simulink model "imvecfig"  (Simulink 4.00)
settings: Solver=ode45  StartTime=0.0  StopTime=10.0  RelTol=1e-3
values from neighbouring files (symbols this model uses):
  fr0 = [phidr phiqr]    [imdef0vec.m]    (also in imdef1vec.m; imdefrotflux.m = sqrt(phidr^2+phiqr^2); imdefSIvec1.m)
  fs0 = fs    [calc0.m]    (also in imdef0vec.m = [phids phiqs]; imdef1vec.m = [phids phiqs]; imdefrotflux.m = [fs0d fs0q]; imdefSIvec1.m = [phids phiqs])
  Lm = eval(get(hLm,'String'))    [im3d.m]    (also in IMabc2.m = 4.5; imabcparam.m = 0.0847; IMabcrun0.m = 0.0847; IMabcrun1.m = 0.0847)
  p = cos(beta-alpha)    [abcRwdg.m]    (also in alternator.m = 0:pi/20:2*pi; altwdgs.m = 0:pi/20:2*pi; brushlessdcB.m = 0:pi/100:2*pi; brushlessdcnew.m = 0:pi/100:2*pi)
  Rr = input('Rotor resistance)[default = 2] =')    [Actac.m]    (also in im1phase.m = 0.3; im3d.m = eval(get(hRr,'String')); IMabc2.m = 0.02; imabcparam.m = 0.408)
  Rs = eval(get(hRs,'String'))    [im3d.m]    (also in IMabc2.m = 0.01; imabcparam.m = 0.531; IMabcrun0.m = 0.531; IMabcrun1.m = 0.531)
undefined symbols (not defined in the file or in its folder): Gm, Gr, Gs
libraries: simulink3 x1

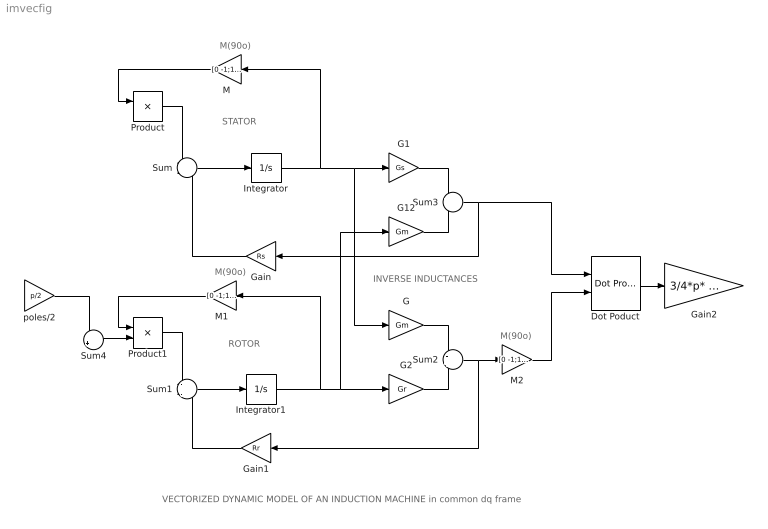
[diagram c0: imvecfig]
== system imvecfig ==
  note: ROTOR
  note: STATOR
  note: VECTORIZED DYNAMIC MODEL OF AN INDUCTION MACHINE in common dq frame
  note: INVERSE INDUCTANCES
  note: M(90o)
  note: M(90o)
  note: M(90o)
  Dot Poduct : simulink3/Math/Dot Product
  G : Gain  Gain=Gm  Multiplication=Element-wise(K.*u)  SaturateOnIntegerOverflow=on
  G1 : Gain  Gain=Gs  Multiplication=Element-wise(K.*u)  SaturateOnIntegerOverflow=on
  G12 : Gain  Gain=Gm  Multiplication=Element-wise(K.*u)  SaturateOnIntegerOverflow=on
  G2 : Gain  Gain=Gr  Multiplication=Element-wise(K.*u)  SaturateOnIntegerOverflow=on
  Gain : Gain  Orientation=left  Gain=Rs  Multiplication=Element-wise(K.*u)  SaturateOnIntegerOverflow=on
  Gain1 : Gain  Orientation=left  Gain=Rr  Multiplication=Element-wise(K.*u)  SaturateOnIntegerOverflow=on
  Gain2 : Gain  Gain=3/4*p* Lm  Multiplication=Element-wise(K.*u)  SaturateOnIntegerOverflow=on
  Integrator : Integrator  ExternalReset=none  InitialConditionSource=internal  InitialCondition=fs0  LimitOutput=off  UpperSaturationLimit=inf  LowerSaturationLimit=-inf  ShowSaturationPort=off  ShowStatePort=off  AbsoluteTolerance=auto
  Integrator1 : Integrator  ExternalReset=none  InitialConditionSource=internal  InitialCondition=fr0  LimitOutput=off  UpperSaturationLimit=inf  LowerSaturationLimit=-inf  ShowSaturationPort=off  ShowStatePort=off  AbsoluteTolerance=auto
  M : Gain  Orientation=left  Gain=[0 -1;1 0]  Multiplication=Matrix(K*u)  SaturateOnIntegerOverflow=on
  M1 : Gain  Orientation=left  Gain=[0 -1;1 0]  Multiplication=Matrix(K*u)  SaturateOnIntegerOverflow=on
  M2 : Gain  Gain=[0 -1;1 0]  Multiplication=Matrix(K*u)  SaturateOnIntegerOverflow=on
  Product : Product  Inputs=2  Multiplication=Element-wise(.*)  SaturateOnIntegerOverflow=on
  Product1 : Product  Inputs=2  Multiplication=Element-wise(.*)  SaturateOnIntegerOverflow=on
  Sum : Sum  Inputs=-+-  SaturateOnIntegerOverflow=on
  Sum1 : Sum  Inputs=-+-  SaturateOnIntegerOverflow=on
  Sum2 : Sum  Inputs=-+  SaturateOnIntegerOverflow=on
  Sum3 : Sum  Inputs=+-  SaturateOnIntegerOverflow=on
  Sum4 : Sum  Inputs=-+|  SaturateOnIntegerOverflow=on
  poles/2 : Gain  Gain=p/2  Multiplication=Element-wise(K.*u)  SaturateOnIntegerOverflow=on
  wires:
  ? -> Sum1/2
  Gain1/1 -> Sum1/3
  Integrator/1 -> M/1, G1/1, G/1
  Integrator1/1 -> M1/1, G2/1, G12/1
  Product1/1 -> Sum1/1
  M1/1 -> Product1/1
  Product/1 -> Sum/1
  M/1 -> Product/1
  Sum4/1 -> Product1/2
  ? -> Product/2, Sum4/2
  Sum1/1 -> Integrator1/1
  Sum/1 -> Integrator/1
  ? -> poles/2/1
  G1/1 -> Sum3/1
  G12/1 -> Sum3/2
  Sum3/1 -> Dot Poduct/1, Gain/1
  G/1 -> Sum2/1
  G2/1 -> Sum2/2
  Sum2/1 -> M2/1, Gain1/1
  Gain/1 -> Sum/3
  M2/1 -> Dot Poduct/2
  Dot Poduct/1 -> Gain2/1
  poles/2/1 -> Sum4/1
  ? -> Sum/2
  Gain2/1 -> ?
